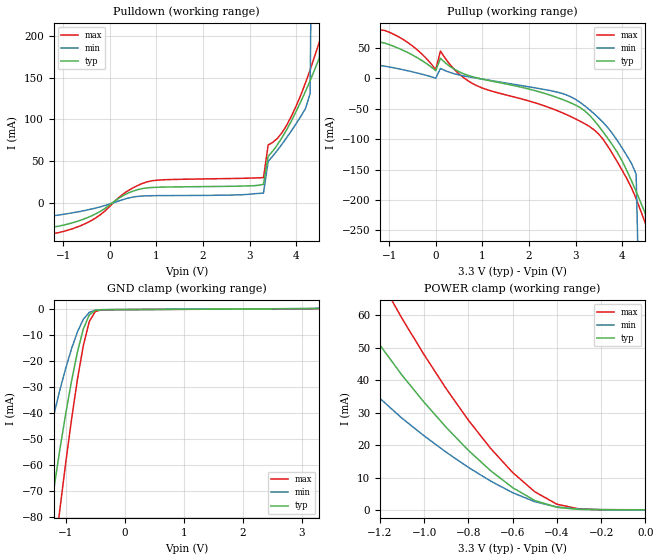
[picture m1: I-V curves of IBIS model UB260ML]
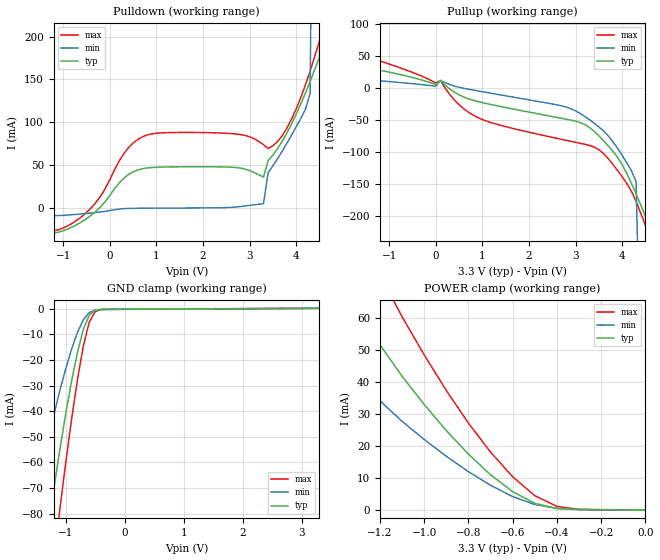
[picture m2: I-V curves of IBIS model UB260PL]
| IBIS file ub260oml.ibs created by s2ibis2 version 1.1
| North Carolina State University Electronics Research Laboratory  1995
[IBIS ver]   2.1
[File name]   z6usb11l.ibs
[File Rev]   1.0
[Date]   Tuesday, April 23, 2002
[Source]   From silicon level SPICE at TOSHIBA.
[Notes]   This model does not include the values of Package Model
[Disclaimer]   None.
[Copyright]   Copyright(C) TOSHIBA Corp. 1996-1998. All Rights Reserved
|   Component TC260C
[Component]   TC260C
[Manufacturer]   TOSHIBA
[Package]
| variable   typ   min   max
R_pkg   1.0000f   NA   NA
L_pkg   1.0000fH   NA   NA
C_pkg   1.0000fF   NA   NA
[Pin]  signal_name   model_name   R_pin   L_pin   C_pin
DM   DM   UB260ML
DP   DP   UB260PL
VDDS   VDDS   POWER
VSS   VSS   GND
| Models and submodels in the file (2): UB260ML (3-state), UB260PL (3-state)
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|   Model UB260ML
[Model]   UB260ML
Model_type   3-state
Polarity   Non-Inverting
C_comp   7.964pF   NA   NA
|Variable   typ   min   max
[Voltage range]  3.3   3.0   3.6
[Temperature Range]   25.0000   100.0000   0.000
[Pullup Reference]   3.3000V   3.0000V   3.6000V
[Pulldown Reference]   0.000V   0.000V   0.000V
[POWER Clamp Reference]   3.3000V   3.0000V   3.6000V
[GND Clamp Reference]   0.000V   0.000V   0.000V
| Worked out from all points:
|   slope of the pulldown table from 0 to 0.495 V, typ, clamps not added: 30.4 ohm
|   slope of the pullup table from 0 to 0.495 V, typ, clamps not added: 312 ohm
|   GND clamp passes 1 mA (typ) near -0.52 V on its own axis
|   POWER clamp passes 1 mA (typ) near -0.41 V on its own axis
[Pulldown]
| voltage   I(typ)   I(min)   I(max)
-3.3V     -3.54mA    -1.53mA    -7.91mA
-1.7V     -5.158mA   -3.407mA   -7.509mA
-1.3V     -29.18mA   -15.67mA   -37.04mA
800mV     18.2mA     8.715mA    25.44mA
3.3V      22.36mA    12mA       30.47mA
3.4V      55.92mA    49.93mA    69.48mA
3.8V      87.97mA    78.44mA    93.38mA
4.2V      133.5mA    112.9mA    143.6mA
4.3V      146.2mA    130.5mA    159.1mA
4.5V      173.5mA    1.253A     192.7mA
4.7V      637.2mA    5.063A     229.7mA
6.6V      45.4A      50.85A     38.79A
[Pullup]
| voltage   I(typ)   I(min)   I(max)
-3.3V     -13.43mA   -3.74mA    -77.68mA
-1.5V     23.34mA    7.04mA     21.12mA
-1.3V     60.83mA    22.11mA    80.22mA
-1.1V     57.79mA    19.85mA    78.52mA
0V        12.38mA    -36.87uA   14.16mA
100mV     32.76mA    16.11mA    44.71mA
800mV     2.22mA     1.081mA    -9.172mA
2.9V      -40.63mA   -30.66mA   -63.14mA
4.2V      -168.5mA   -139.9mA   -180mA
4.5V      -222.9mA   -807.3mA   -238.6mA
4.7V      -483.8mA   -3.042A    -282.4mA
6.6V      -26.71A    -29.96A    -22.77A
[GND_clamp]
| voltage   I(typ)   I(min)   I(max)
-3.3V     -26.62A    -25.55A    -26.99A
-1.4V     -356.8mA   -160.3mA   -479.8mA
-1.3V     -95.09mA   -55.74mA   -129.5mA
-1.2V     -69.39mA   -40.75mA   -96.7mA
-1.1V     -54.4mA    -31.41mA   -77.57mA
-900mV    -27.78mA   -15.34mA   -42.49mA
-800mV    -16.59mA   -8.835mA   -27.11mA
-700mV    -7.701mA   -3.996mA   -14.1mA
-600mV    -2.328mA   -1.35mA    -4.928mA
-500mV    -587.6uA   -485.2uA   -1.043mA
-400mV    -332.4uA   -312.2uA   -385.5uA
3.3V      125.4uA    325.2uA    101.4uA
[POWER_clamp]
| voltage   I(typ)   I(min)   I(max)
-3.3V     45.19A     43.36A     45.82A
-1.4V     532.1mA    217.5mA    733.1mA
-1.3V     78.89mA    49.47mA    109.4mA
-1.2V     50.88mA    34.47mA    71.25mA
-1.1V     41.61mA    28.34mA    59.1mA
-900mV    25.5mA     17.85mA    37.41mA
-800mV    18.45mA    13.19mA    27.75mA
-600mV    6.945mA    5.392mA    11.62mA
-500mV    2.994mA    2.631mA    5.681mA
-400mV    883.9uA    999.3uA    1.844mA
-300mV    246.7uA    325.2uA    406uA
0V        125.4uA    114uA      136.8uA
[Ramp]
| variable   typ   min   max
dV/dt_r   1.5128/0.1869u   1.1450/0.1913u   1.7317/0.1855u
dV/dt_f   1.4464/0.2033u   1.0280/0.2098u   1.6831/0.2050u
R_load = 50.0000
| End [Model] UB260ML
|   Model UB260PL
[Model]   UB260PL
Model_type   3-state
Polarity   Non-Inverting
C_comp   7.914pF   NA   NA
|Variable   typ   min   max
[Voltage range]  3.3   3.0   3.6
[Temperature Range]   25.0000   100.0000   0.000
[Pullup Reference]   3.3000V   3.0000V   3.6000V
[Pulldown Reference]   0.000V   0.000V   0.000V
[POWER Clamp Reference]   3.3000V   3.0000V   3.6000V
[GND Clamp Reference]   0.000V   0.000V   0.000V
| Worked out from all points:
|   slope of the pulldown table from 0 to 0.495 V, typ, clamps not added: 18.1 ohm
|   slope of the pullup table from 0 to 0.495 V, typ, clamps not added: 31.2 ohm
|   GND clamp passes 1 mA (typ) near -0.52 V on its own axis
|   POWER clamp passes 1 mA (typ) near -0.43 V on its own axis
[Pulldown]
| voltage   I(typ)   I(min)   I(max)
-3.3V     17.28mA    -3.78mA    43.96mA
-1.7V     10.47mA    -4.295mA   28.76mA
-1.5V     1.814mA    -6.215mA   18.65mA
-1.3V     -30.44mA   -9.479mA   -27.67mA
-400mV    -8.694mA   -6.015mA   -98.28uA
700mV     45.75mA    -432.1uA   82.9mA
3.3V      35.98mA    4.868mA    73.71mA
3.4V      55.32mA    41.22mA    69.39mA
4.2V      134.1mA    115mA      143.6mA
4.5V      176mA      1.243A     194.7mA
4.7V      638.8mA    5.05A      233.3mA
6.6V      45.4A      50.81A     38.79A
[Pullup]
| voltage   I(typ)   I(min)   I(max)
-3.3V     41.26mA    12.74mA    92.67mA
-2.1V     15.51mA    5.68mA     34.41mA
-1.3V     29.26mA    12.23mA    44.61mA
100mV     12.1mA     12.48mA    12.2mA
900mV     -20.51mA   -3.978mA   -45.57mA
2.8V      -48.22mA   -29.29mA   -81.17mA
3.5V      -74.13mA   -60.21mA   -95.74mA
4.1V      -133.1mA   -116.3mA   -148.4mA
4.3V      -164.9mA   -146.1mA   -176.4mA
4.5V      -199.9mA   -802.5mA   -214mA
4.7V      -469mA     -3.041A    -255.5mA
6.6V      -26.71A    -29.97A    -22.77A
[GND_clamp]
| voltage   I(typ)   I(min)   I(max)
-3.3V     -26.62A    -25.55A    -26.99A
-1.4V     -357.4mA   -161.1mA   -480.5mA
-1.3V     -96.11mA   -56.64mA   -130.8mA
-1.2V     -70.33mA   -41.57mA   -97.86mA
-1.1V     -55.24mA   -32.13mA   -78.61mA
-900mV    -28.42mA   -15.89mA   -43.29mA
-800mV    -17.12mA   -9.298mA   -27.79mA
-700mV    -8.101mA   -4.347mA   -14.64mA
-600mV    -2.557mA   -1.548mA   -5.283mA
-500mV    -648.3uA   -546.4uA   -1.169mA
-400mV    -339uA     -322.4uA   -399.9uA
3.3V      125.4uA    209.9uA    101.4uA
[POWER_clamp]
| voltage   I(typ)   I(min)   I(max)
-3.3V     45.19A     43.36A     45.82A
-1.4V     533.1mA    217.8mA    734.7mA
-1.3V     80.31mA    49.56mA    112.4mA
-1.2V     51.76mA    34.25mA    73.55mA
-1.1V     41.94mA    27.82mA    60.57mA
-900mV    24.93mA    16.88mA    37.47mA
-800mV    17.55mA    12.07mA    27.26mA
-600mV    5.799mA    4.262mA    10.46mA
-500mV    2.138mA    1.783mA    4.552mA
-400mV    518.8uA    560.7uA    1.19mA
-300mV    191.2uA    209.9uA    265.4uA
0V        125.4uA    114uA      136.8uA
[Ramp]
| variable   typ   min   max
dV/dt_r   1.5130/0.1885u   1.1602/0.1959u   1.7318/0.1867u
dV/dt_f   1.4463/0.2032u   1.0276/0.2097u   1.6831/0.2049u
R_load = 50.0000
| End [Model] UB260PL
| End [Component] TC260C
